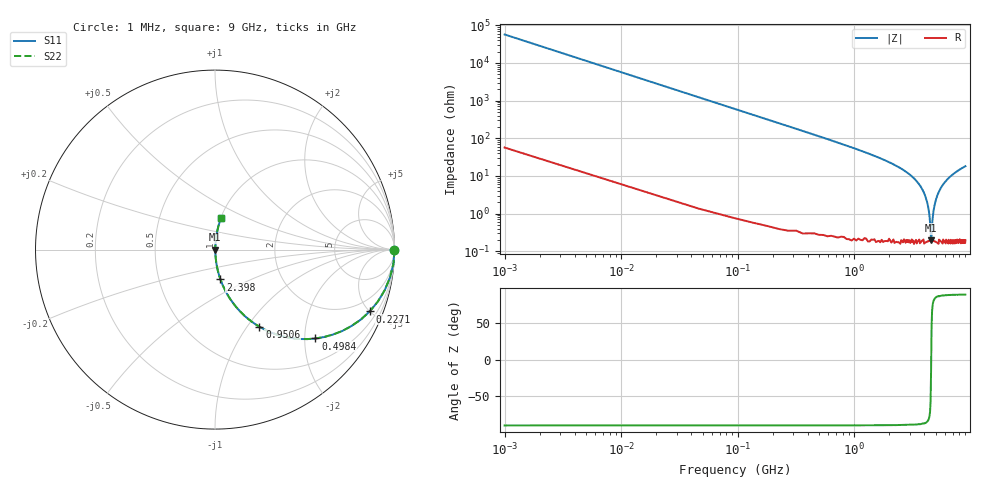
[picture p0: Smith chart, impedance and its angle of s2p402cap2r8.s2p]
! AVX Thin Film Operation		Date: December 2010
! Description: Accu-P® Series, Thin Film, SMD, RF Capacitor
! Part Number: 04021J2R8ABS
! 50 MHz  -  9 GHz
! Serial Measurements
# MHZ S MA R 50
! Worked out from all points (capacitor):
!   200 points, 1 MHz to 9 GHz, reference 50 ohm
!   read as one part in series: C = 2.8 pF near 46.22 MHz
!   lowest |Z| = 197 mohm at 4.568 GHz (marker M1)
!   series resonance near 4.578 GHz, so ESL is about 430 pH
!   S11 on the Smith chart (normalised r, x): 1 MHz: open; 227.1 MHz: 1.01, -4.99; 498.4 MHz: 1.01, -2.25; 950.6 MHz: 1.00, -1.14; 2.398 GHz: 1.00, -0.34; 9 GHz: 1.00, +0.36
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1  1 -0.1  0.001759 89.8  0.001759 89.8  1 -0.1
46.221  0.997 -4.6  0.081 85.3  0.081 85.3  0.997 -4.6
91.442  0.987 -9.1  0.159 80.8  0.159 80.8  0.987 -9.1
136.663  0.972 -13.5  0.234 76.4  0.234 76.4  0.972 -13.5
227.106  0.928 -21.8  0.372 68.1  0.372 68.1  0.928 -21.8
498.432  0.747 -41.5  0.663 48.3  0.663 48.3  0.747 -41.5
950.643  0.496 -60.1  0.867 29.7  0.867 29.7  0.496 -60.1
1538.518  0.311 -71.5  0.949 18.1  0.949 18.1  0.311 -71.5
2397.719  0.169 -79.6  0.984 9.7  0.984 9.7  0.169 -79.6
3030.814  0.105 -83.0  0.993 6.0  0.993 6.0  0.105 -83.0
3709.131  0.053 -85.0  0.997 3.0  0.997 3.0  0.053 -85.0
4161.342  0.024 -84.3  0.998 1.4  0.998 1.4  0.024 -84.3
4387.447  0.011 -79.7  0.998 0.6  0.998 0.6  0.011 -79.7
4477.889  0.005774 -71.6  0.998 0.3  0.998 0.3  0.005774 -71.6
4523.111  0.003494 -58.9  0.998 0.2  0.998 0.2  0.003494 -58.9
4568.332  0.001873 -16.4  0.998 0.0  0.998 0.0  0.001873 -16.4
4749.216  0.009272 78.3  0.998 -0.5  0.998 -0.5  0.009272 78.3
4975.322  0.021 83.8  0.998 -1.2  0.998 -1.2  0.021 83.8
5517.975  0.047 85.1  0.997 -2.7  0.997 -2.7  0.047 85.1
6015.407  0.068 84.6  0.996 -3.9  0.996 -3.9  0.068 84.6
7507.704  0.127 81.9  0.99 -7.3  0.99 -7.3  0.127 81.9
9000  0.178 79.2  0.982 -10.2  0.982 -10.2  0.178 79.2
